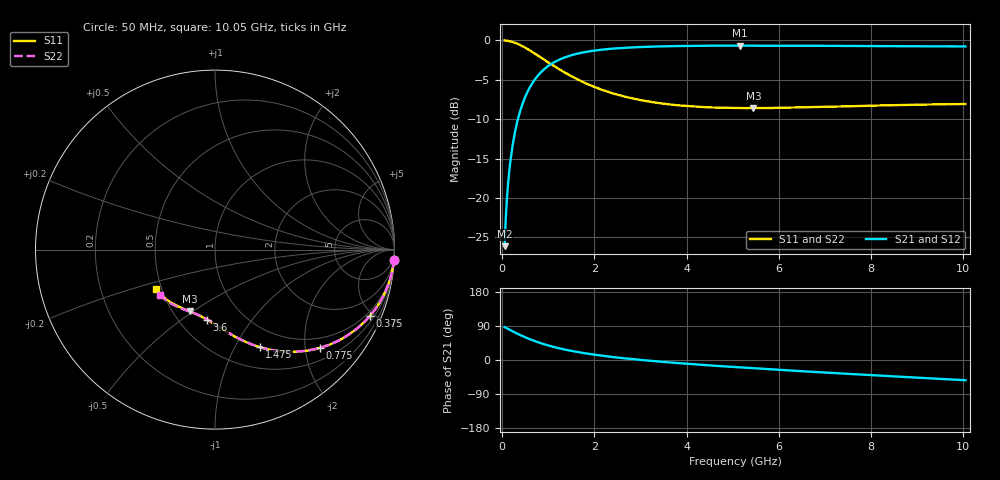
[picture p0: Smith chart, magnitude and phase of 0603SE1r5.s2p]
! AVX Thin Film Operation		Date: August 2001
! Description: Accu-P® Series, Thin Film, SMD, RF Capacitor
! Part Number: 06035J1R5ABT
! 50 MHz  -  10.05 GHz
! Serial Measurements
# mhz S db R 50
!	S11		S21		S12		S22
!	dB	Phase	dB	Phase	dB	Phase	dB	Phase
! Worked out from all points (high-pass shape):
!   401 points, 50 MHz to 10.05 GHz, reference 50 ohm
!   highest |S21| = -0.66 dB at 5.15 GHz (marker M1); lowest = -26.1 dB at 50 MHz (marker M2)
!   |S21| within 3 dB of the highest: 907.6 MHz to end of sweep
!   lowest |S11| = -8.6 dB at 5.45 GHz (marker M3), VSWR 2.18, Z = 30.3 - j24.3 ohm
!   |S11| at or under -10 dB: nowhere
!   |S22| runs from -8.6 to 0.0 dB; largest |S21 - S12| = 0
!   S11 on the Smith chart (normalised r, x): 50 MHz: 1, -35; 375 MHz: 0.76, -4.72; 775 MHz: 0.76, -2.32; 1.475 GHz: 0.75, -1.26; 3.6 GHz: 0.68, -0.63; 10.05 GHz: 0.47, -0.25
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50  -0.01 -3.2  -26.10 86.8  -26.10 86.8  -0.01 -3.2
75  -0.02 -4.9  -22.61 85.2  -22.61 85.2  -0.02 -4.9
125  -0.07 -8.1  -18.19 82.0  -18.19 82.0  -0.07 -8.1
175  -0.13 -11.3  -15.35 78.7  -15.35 78.7  -0.13 -11.3
225  -0.21 -14.4  -13.27 75.6  -13.27 75.6  -0.21 -14.4
275  -0.31 -17.5  -11.64 72.5  -11.64 72.5  -0.31 -17.5
375  -0.55 -23.3  -9.22 66.7  -9.22 66.7  -0.55 -23.3
550  -1.10 -32.8  -6.49 57.1  -6.49 57.1  -1.10 -32.8
775  -1.93 -43.2  -4.45 46.8  -4.45 46.8  -1.93 -43.2
1100  -3.18 -55.1  -2.85 34.9  -2.85 34.9  -3.18 -55.1
1475  -4.47 -65.4  -1.92 24.6  -1.92 24.6  -4.47 -65.3
1725  -5.21 -70.9  -1.56 19.1  -1.56 19.1  -5.21 -70.7
2025  -5.96 -76.3  -1.27 13.7  -1.27 13.7  -5.96 -76.2
2425  -6.76 -82.5  -1.04 7.5  -1.04 7.5  -6.76 -82.2
3400  -7.96 -94.3  -0.77 -4.0  -0.77 -4.0  -7.95 -93.5
3600  -8.10 -96.3  -0.74 -6.1  -0.74 -6.1  -8.09 -95.5
5050  -8.58 -109.6  -0.66 -18.7  -0.66 -18.7  -8.56 -107.6
5150  -8.58 -110.0  -0.66 -19.5  -0.66 -19.5  -8.57 -108.8
5450  -8.59 -112.2  -0.66 -21.9  -0.66 -21.9  -8.57 -110.2
6725  -8.48 -122.4  -0.69 -31.1  -0.69 -31.1  -8.46 -119.4
8400  -8.23 -134.2  -0.73 -42.5  -0.73 -42.5  -8.20 -130.2
10050  -8.08 -145.8  -0.77 -53.4  -0.77 -53.4  -8.04 -140.4
